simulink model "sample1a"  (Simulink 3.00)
settings: Solver=ode5  StartTime=0.0  StopTime=200  FixedStep=0.5  MaxStep=0.5  RelTol=1e-3  AbsTol=1e-3
libraries: simulink_extras x1

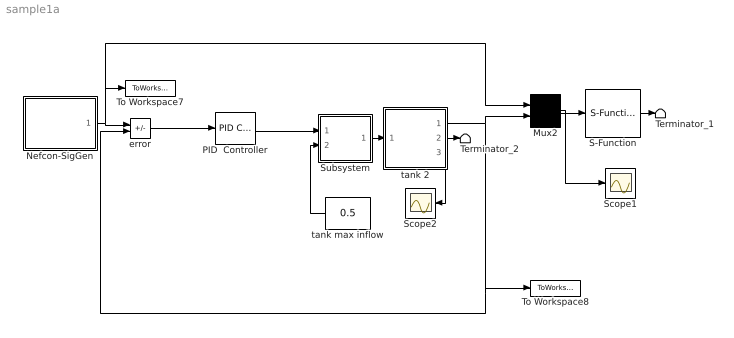
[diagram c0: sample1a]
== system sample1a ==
  Mux2 : Mux  Inputs=2
  Nefcon-SigGen : Subsystem
  PID  Controller : simulink_extras/Additional Linear/PID Controller  P=2  I=0  D=1
  S-Function : S-Function  FunctionName=animtank  Parameters=1  PortCounts=[]  SFunctionModules=''
  Scope1 : Scope
  Scope2 : Scope
  Subsystem : Subsystem  mask(Valve){}
      mask help: Valve
      mask init:
      | InitialPosition = @1;
  Terminator_1 : Terminator
  Terminator_2 : Terminator
  To Workspace7 : ToWorkspace  VariableName=u  SampleTime=0  SaveFormat=Matrix
  To Workspace8 : ToWorkspace  VariableName=y  SampleTime=0  SaveFormat=Matrix
  error : Sum  Inputs=+-  SaturateOnIntegerOverflow=on
  tank 2 : Subsystem  mask(Water tank){}
      mask help: Cylindrical water tank with overflow signal
      mask init:
      | ht=@1;area=@2;outletArea=@3;overflowLimit=@4;initialHt=@5;
  tank max inflow : Constant  Orientation=left  Value=0.5
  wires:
  error/1 -> PID  Controller/1
  tank 2/3(overflow flag) -> Scope2/1
  Mux2/1 -> Scope1/1, S-Function/1
  Subsystem/1(out flow) -> tank 2/1(flow in)
  tank max inflow/1 -> Subsystem/2(source flow)
  Nefcon-SigGen/1(out_1) -> error/1, Mux2/1, To Workspace7/1
  PID  Controller/1 -> Subsystem/1(control)
  tank 2/1(water level) -> error/2, To Workspace8/1, Mux2/2
  S-Function/1 -> Terminator_1/1
  tank 2/2(flow out) -> Terminator_2/1

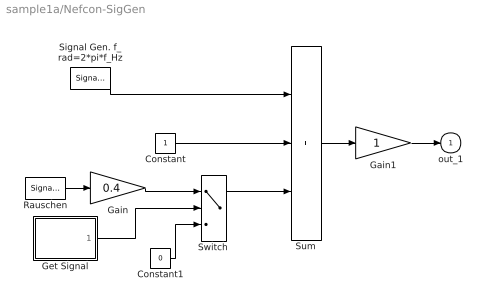
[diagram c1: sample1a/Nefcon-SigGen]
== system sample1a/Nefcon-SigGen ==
  Constant : Constant  Value=1
  Constant1 : Constant  Value=0
  Gain : Gain  Gain=0.4  SaturateOnIntegerOverflow=on
  Gain1 : Gain  Gain=1  SaturateOnIntegerOverflow=on
  Get Signal : Subsystem  mask(GEt Signal){}
      mask help: Put a signal into the MATLAB workspace. Specify the signal width and name.
      mask init:
      | width=@1;name=@2;
  Rauschen : SignalGenerator  WaveForm=random  Amplitude=1.000000  Frequency=1.000000  Units=rad/sec
  Signal Gen. f_rad=2*pi*f_Hz : SignalGenerator  WaveForm=square  Amplitude=0.500000  Frequency=0.050000  Units=rad/sec
  Sum : Sum  Inputs=+++  SaturateOnIntegerOverflow=on
  Switch : Switch  Threshold=0.5
  out_1 : Outport  Port=1
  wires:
  Constant/1 -> Sum/2
  Rauschen/1 -> Gain/1
  Signal Gen. f_rad=2*pi*f_Hz/1 -> Sum/1
  Gain1/1 -> out_1/1
  Sum/1 -> Gain1/1
  Switch/1 -> Sum/3
  Gain/1 -> Switch/1
  Constant1/1 -> Switch/3
  Get Signal/1(out_1) -> Switch/2

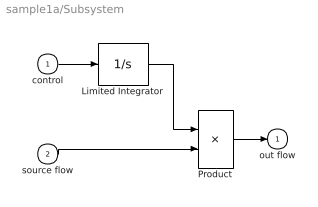
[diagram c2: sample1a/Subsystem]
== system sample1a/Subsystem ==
  control : Inport  Port=1  PortWidth=-1  SampleTime=-1  DataType=auto
  source flow : Inport  Port=2  PortWidth=-1  SampleTime=-1  DataType=auto
  Limited Integrator : Integrator  ExternalReset=none  InitialConditionSource=internal  InitialCondition=InitialPosition  LimitOutput=on  UpperSaturationLimit=1  LowerSaturationLimit=0  ShowSaturationPort=off  ShowStatePort=off  AbsoluteTolerance=auto
  Product : Product  Inputs=2  SaturateOnIntegerOverflow=on
  out flow : Outport  Port=1
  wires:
  Limited Integrator/1 -> Product/1
  control/1 -> Limited Integrator/1
  Product/1 -> out flow/1
  source flow/1 -> Product/2

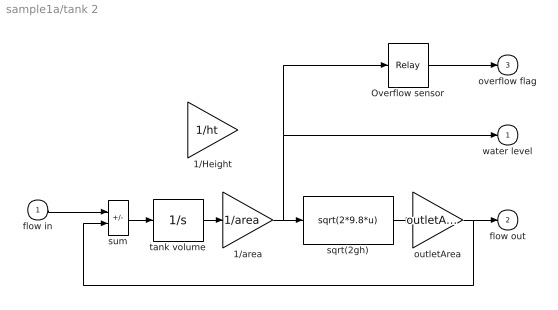
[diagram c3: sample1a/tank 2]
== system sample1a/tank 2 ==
  flow in : Inport  Port=1  PortWidth=-1  SampleTime=-1  DataType=auto
  1/Height : Gain  Gain=1/ht  SaturateOnIntegerOverflow=on
  1/area : Gain  Gain=1/area  SaturateOnIntegerOverflow=on
  Overflow sensor : Relay  OnSwitchValue=ht - overflowLimit  OffSwitchValue=ht - overflowLimit  OnOutputValue=1  OffOutputValue=0
  outletArea : Gain  Gain=outletArea  SaturateOnIntegerOverflow=on
  sqrt(2gh) : Fcn  Expr=sqrt(2*9.8*u)
  sum : Sum  Inputs=+-  SaturateOnIntegerOverflow=on
  tank volume : Integrator  ExternalReset=none  InitialConditionSource=internal  InitialCondition=initialHt * area  LimitOutput=on  UpperSaturationLimit=ht * area  LowerSaturationLimit=0  ShowSaturationPort=off  ShowStatePort=off  AbsoluteTolerance=auto
  water level : Outport  Port=1
  flow out : Outport  Port=2
  overflow flag : Outport  Port=3
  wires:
  sum/1 -> tank volume/1
  flow in/1 -> sum/1
  Overflow sensor/1 -> overflow flag/1
  tank volume/1 -> 1/area/1
  sqrt(2gh)/1 -> outletArea/1
  outletArea/1 -> flow out/1, sum/2
  1/area/1 -> sqrt(2gh)/1, Overflow sensor/1, water level/1

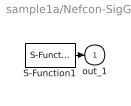
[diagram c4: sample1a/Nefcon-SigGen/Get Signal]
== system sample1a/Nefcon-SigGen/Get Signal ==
  S-Function1 : S-Function  FunctionName=getsig  Parameters=width,name  PortCounts=[]  SFunctionModules=''
  out_1 : Outport  Port=1
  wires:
  S-Function1/1 -> out_1/1
